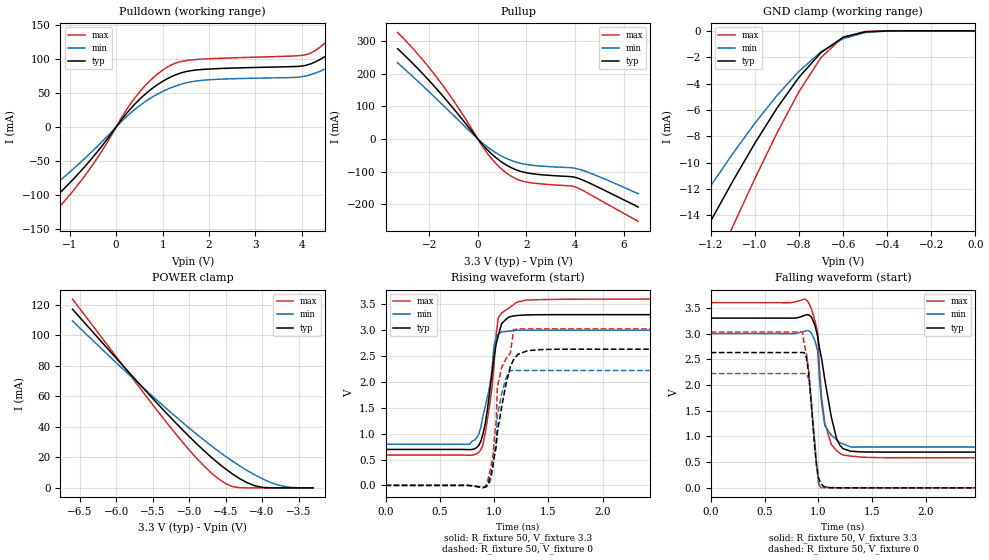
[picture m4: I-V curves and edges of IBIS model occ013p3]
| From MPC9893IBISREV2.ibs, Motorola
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|  Output Buffer at 3.3V Application
[Model]   occ013p3
Model_type   Output
Enable   Active-Low
Polarity   Non-Inverting
Vref=1.5
Cref=1pf
Rref=50
| Variable   typ   min   max
C_comp   5p   5p   5p
[Temperature Range]   27.00   100.00   -45.00
[Voltage Range]   3.30V   3.00V   3.60V
[Pulldown Reference]   0.000V   0.000V   0.000V
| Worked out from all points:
|   slope of the pulldown table from 0 to 0.495 V, typ, clamps not added: 12.4 ohm
|   slope of the pullup table from 0 to 0.495 V, typ, clamps not added: 12.1 ohm
|   GND clamp passes 1 mA (typ) near -0.64 V on its own axis
|   POWER clamp passes 1 mA (typ) near -4.06 V on its own axis
|   rising waveform, R_fixture 50, V_fixture 3.3: 20-80 % time 105ps typ, 105ps min, 91.8ps max; typ from 0.695 V to 3.3 V
|   falling waveform, R_fixture 50, V_fixture 3.3: 20-80 % time 133ps typ, 61.6ps min, 76.5ps max; typ from 3.3 V to 0.695 V
|   rising waveform, R_fixture 50, V_fixture 0: 20-80 % time 127ps typ, 77.6ps min, 112ps max; typ from 0 V to 2.63 V
|   falling waveform, R_fixture 50, V_fixture 0: 20-80 % time 63.4ps typ, 54ps min, 76.3ps max; typ from 2.63 V to 0 V
[Pulldown]
|Voltage   I(typ)   I(min)   I(max)
-3.3V     -209.8mA   -184.1mA   -233.1mA
-2.5V     -171.4mA   -145.7mA   -196.3mA
-2V       -144.6mA   -120.9mA   -169.9mA
-1.6V     -121.3mA   -100.1mA   -144.4mA
-600mV    -52.28mA   -41.26mA   -64.61mA
500mV     40.26mA    30.94mA    50.94mA
1.2V      74.05mA    58.02mA    91.38mA
4.1V      90.56mA    75mA       106.1mA
4.8V      118.5mA    95.76mA    145.2mA
5.2V      146.1mA    114.5mA    186.5mA
5.7V      200mA      148.6mA    270.9mA
6.6V      419.9mA    278.5mA    628.6mA
[Pullup]
|Voltage   I(typ)   I(min)   I(max)
-3.3V     276.2mA    233mA      325.6mA
-2.5V     217.6mA    178.8mA    262.3mA
-1.7V     153.4mA    122.6mA    189.2mA
-800mV    74.59mA    57.3mA     95.02mA
300mV     -26.06mA   -19.2mA    -34.48mA
700mV     -54.72mA   -40.53mA   -71.91mA
1.1V      -76.73mA   -57.15mA   -100.1mA
1.5V      -92.4mA    -69.23mA   -119.7mA
1.9V      -102.1mA   -76.99mA   -130.5mA
4V        -117.6mA   -89.99mA   -146.7mA
4.8V      -142.5mA   -110mA     -177.7mA
6.6V      -208.6mA   -167.9mA   -252.3mA
[GND_clamp]
|Voltage   I(typ)   I(min)   I(max)
-3.3V     -85.27mA   -74.38mA   -97.87mA
-1.4V     -20.76mA   -16.98mA   -26.15mA
-1.3V     -17.56mA   -14.32mA   -22.34mA
-1.2V     -14.43mA   -11.76mA   -18.57mA
-1.1V     -11.4mA    -9.311mA   -14.84mA
-900mV    -5.871mA   -4.914mA   -7.763mA
-800mV    -3.524mA   -3.07mA    -4.613mA
-700mV    -1.653mA   -1.587mA   -2.027mA
-600mV    -494uA     -597.7uA   -480.9uA
-500mV    -78.44uA   -130.1uA   -51.01uA
-400mV    -7.209uA   -15.25uA   -2.718uA
1.97fV    -33.27pA   -701.5pA   -3.87pA
[POWER_clamp]
|Voltage   I(typ)   I(min)   I(max)
-6.6V     117mA      109.4mA    123.6mA
-5.8V     74.29mA    73.06mA    73.28mA
-5.2V     43.37mA    47.3mA     36.28mA
-4.9V     29.01mA    35.26mA    19.52mA
-4.6V     16.15mA    24.09mA    5.976mA
-4.5V     12.36mA    20.62mA    2.814mA
-4.4V     8.904mA    17.3mA     800.8uA
-4.2V     3.283mA    11.23mA    5.412uA
-4.1V     1.379mA    8.513mA    174.8nA
-3.9V     43.18uA    3.908mA    72.88pA
-3.7V     227.2nA    935.3uA    4.59pA
-3.3V     48.11pA    322.6nA    3.568pA
[Ramp]
dV/dt_r   1.56/105p   1.29/169p   1.81/69.3p
dV/dt_f   1.56/127.4p   1.3/192.1p   1.81/88.1p
R_load = 50
[Rising Waveform]
R_fixture = 50
V_fixture = 3.3
V_fixture_min = 3.0
V_fixture_max = 3.6
|Time (ns) Voltage(typ)  Voltage(min)  Voltage(max)
0s        695mV      795.2mV    585.3mV
776ps     691.2mV    795.2mV    581.3mV
858ps     771.9mV    985.6mV    638mV
895ps     972.8mV    1.315V     766.3mV
958ps     1.778V     1.889V     1.542V
1ns       2.487V     2.722V     2.333V
1.04ns    2.904V     2.926V     3.247V
1.07ns    3.129V     2.965V     3.333V
1.21ns    3.283V     2.998V     3.539V
5ns       3.3V       3V         3.6V
[Falling Waveform]
R_fixture = 50
V_fixture = 3.3
V_fixture_min = 3.0
V_fixture_max = 3.6
|Time (ns) Voltage(typ)  Voltage(min)  Voltage(max)
0s        3.3V       3V         3.6V
908ps     3.368V     3.061V     3.608V
994ps     2.939V     2.654V     3.01V
1.01ns    2.718V     2.137V     2.349V
1.03ns    2.52V      1.654V     1.761V
1.06ns    2.104V     1.21V      1.263V
1.12ns    1.384V     1.023V     846.3mV
1.17ns    950.1mV    937.9mV    721mV
1.23ns    761.7mV    854.5mV    637.3mV
5ns       695mV      795.3mV    585.3mV
[Rising Waveform]
R_fixture = 50
V_fixture = 0
V_fixture_min = 0
V_fixture_max = 0
|Time (ns) Voltage(typ)  Voltage(min)  Voltage(max)
0s        286.8pV    9.073nV    24.07pV
924ps     -30.9mV    -32.03mV   -10.33mV
991ps     416.9mV    374.4mV    591mV
1.02ns    757mV      893.3mV    1.26V
1.03ns    1.015V     1.343V     1.899V
1.11ns    1.961V     2.075V     2.446V
1.15ns    2.296V     2.221V     2.553V
1.18ns    2.432V     2.221V     3.004V
1.43ns    2.625V     2.221V     3.025V
5ns       2.632V     2.221V     3.025V
[Falling Waveform]
R_fixture = 50
V_fixture = 0
V_fixture_min = 0
V_fixture_max = 0
|Time (ns) Voltage(typ)  Voltage(min)  Voltage(max)
0s        2.63V      2.222V     3.03V
853ps     2.63V      2.222V     3.03V
890ps     2.524V     2.217V     2.597V
919ps     2.025V     1.996V     2.099V
966ps     783.7mV    921.9mV    881.6mV
982ps     456.5mV    459.8mV    514.4mV
1ns       209.4mV    107mV      137.6mV
1.02ns    95.09mV    4.92mV     24.83mV
1.1ns     3.325mV    2.05mV     9.039mV
5ns       -11.9uV    304.1nV    11.65uV
